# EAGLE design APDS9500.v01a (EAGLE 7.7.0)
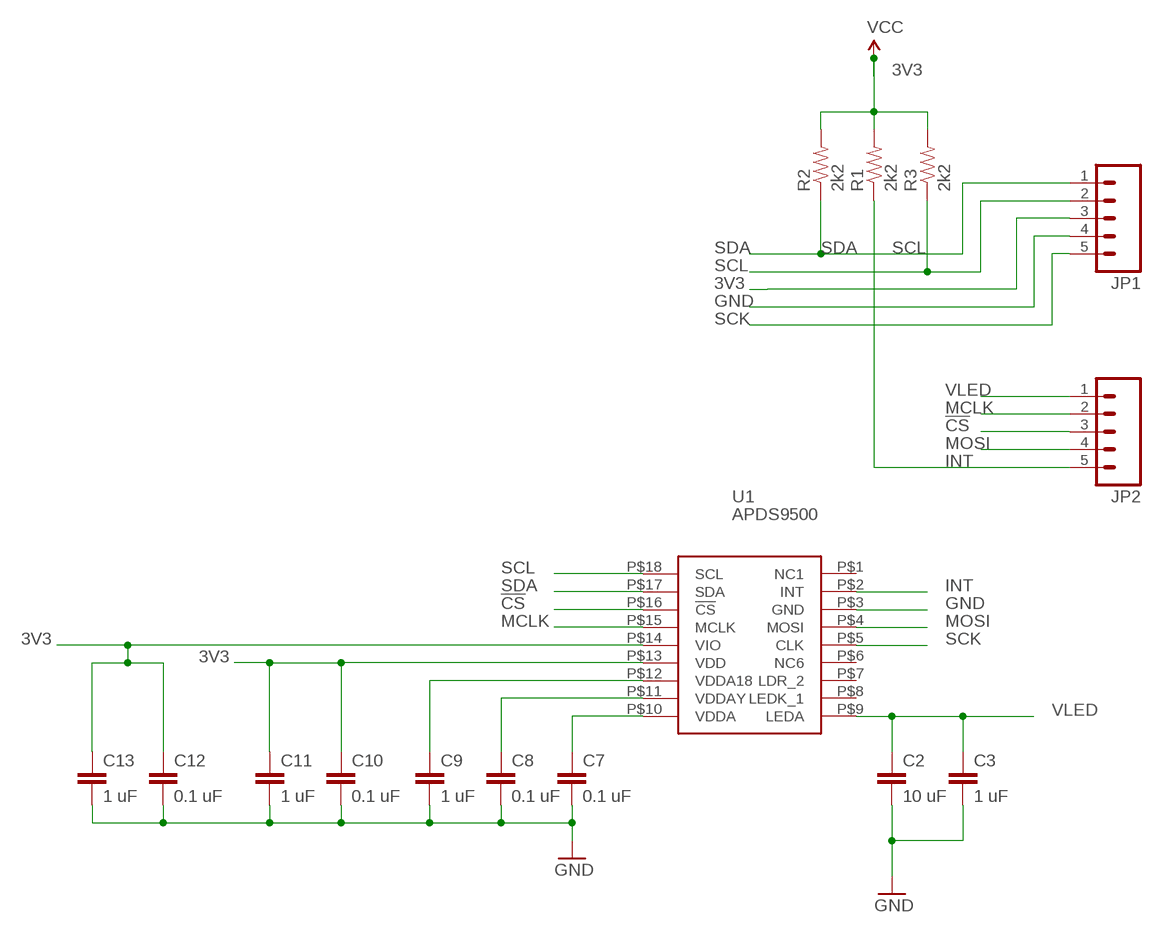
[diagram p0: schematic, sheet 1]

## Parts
C2  10 uF  CAP0402-CAP  [0402-CAP]
C3  1 uF  CAP0402-CAP  [0402-CAP]
C7  0.1 uF  CAP0402-CAP  [0402-CAP]
C8  0.1 uF  CAP0402-CAP  [0402-CAP]
C9  1 uF  CAP0402-CAP  [0402-CAP]
C10  0.1 uF  CAP0402-CAP  [0402-CAP]
C11  1 uF  CAP0402-CAP  [0402-CAP]
C12  0.1 uF  CAP0402-CAP  [0402-CAP]
C13  1 uF  CAP0402-CAP  [0402-CAP]
JP1  M05NO_SILK  [1X05_NO_SILK]
JP2  M05NO_SILK  [1X05_NO_SILK]
R1  2k2  0402RES.KW  [0402-RES]
R2  2k2  0402RES.KW  [0402-RES]
R3  2k2  0402RES.KW  [0402-RES]
U1  APDS9500  [APDS9500]

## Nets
3V3: C10.1 C11.1 C12.1 C13.1 JP1.3 R1.2 R2.2 R3.2 U1.P$13(VDD) U1.P$14(VIO) ; supply symbol labelled VCC
!CS: JP2.3 U1.P$16(!CS)
GND: C2.2 C3.2 C7.2 C8.2 C9.2 C10.2 C11.2 C12.2 C13.2 JP1.4 U1.P$3(GND)
INT: JP2.5 R1.1 U1.P$2(INT)
MCLK: JP2.2 U1.P$15(MCLK)
MOSI: JP2.4 U1.P$4(MOSI)
N$1: C7.1 U1.P$10(VDDA)
N$2: C8.1 U1.P$11(VDDAY)
N$4: C9.1 U1.P$12(VDDA18)
SCK: JP1.5 U1.P$5(CLK)
SCL: JP1.2 R3.1 U1.P$18(SCL)
SDA: JP1.1 R2.1 U1.P$17(SDA)
VLED: C2.1 C3.1 JP2.1 U1.P$9(LEDA)
Unconnected: U1.P$1(NC1) U1.P$6(NC6)

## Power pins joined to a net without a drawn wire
LDR_2: U1.P$7(LDR_2)
LEDK_1: U1.P$8(LEDK_1)

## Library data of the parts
C2 C3 C7-C13 = SparkFun-Capacitors:CAP: Capacitor
JP1 JP2 = SparkFun-Connectors:M05: Header 5 Standard 5-pin 0.1" header. Use with straight break away headers (SKU : PRT-00116), right angle break away headers (PRT-00553), swiss pins (PRT-00743), machine pins (PRT-00117), and female headers (PRT-00115). Molex polarized connector foot print use with SKU : PRT-08230 with associated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
R1-R3 = SparkFun-Resistors:0402RES.KW
U1 = kris:APDS9500: APDS-9500 Broadcom proximity sensor, gesturedetection sensor, camera https://www.broadcom.com/products/optical-sensors/proximity-sensors/apds-9500#overview

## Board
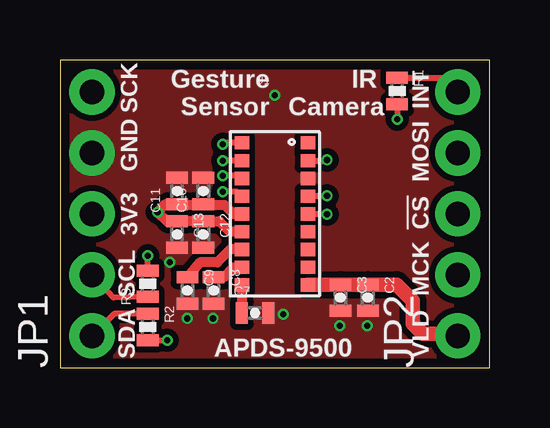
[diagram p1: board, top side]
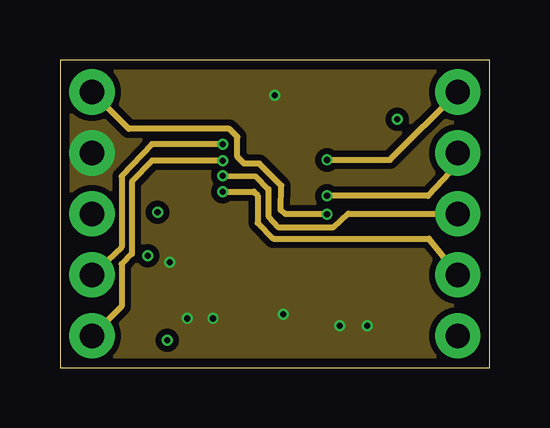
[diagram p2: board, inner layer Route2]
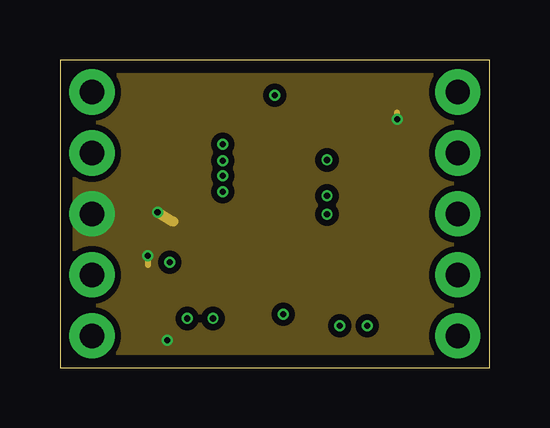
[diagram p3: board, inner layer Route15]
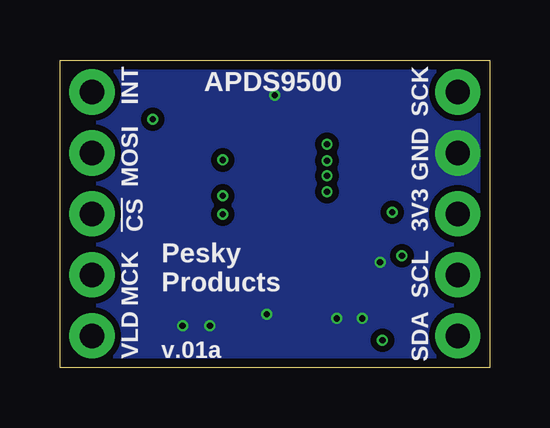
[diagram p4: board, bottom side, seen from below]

Size 17.91 x 12.83 mm. Coordinates in mm from the lower left corner, seen from the top.
Outline: 0,0 17.91,0 17.91,12.83 0,12.83 0,0
Copper layers (1*2*15*16): Top 0.035559375mm / dielectric 0.17018125mm / Route2 0.01778125mm / dielectric 47mil / Route15 0.01778125mm / dielectric 0.17018125mm / Bottom 0.035559375mm
Design rules "OSHPark-4layer *": minimum track width 5mil, minimum drill 10mil, track to track 5mil, track to pad 5mil, pad to pad 5mil, via to via 5mil, smd to smd 5mil, copper to edge 15mil, drill to drill 6mil, minimum pad ring 4mil, minimum via ring 4mil, stop-mask expansion 2.5mil, vias tented up to drill 20mil, thermal gap 10mil

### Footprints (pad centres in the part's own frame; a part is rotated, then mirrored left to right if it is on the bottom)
0402-CAP = smd 0.5 x 0.9: 1 -0.55,0; 2 0.55,0
1X05_NO_SILK = drill 1.016 pad 1.88: 1 0,0; 2 2.54,0; 3 5.08,0; 4 7.62,0; 5 10.16,0
0402-RES = smd 0.5 x 0.9: 1 -0.55,0; 2 0.55,0
APDS9500 = smd 0.6 x 0.55: P$1 1.377,2.96; P$2 1.377,2.22; P$3 1.377,1.48; P$4 1.377,0.74; P$5 1.377,0; P$6 1.377,-0.74; P$7 1.377,-1.48; P$8 1.377,-2.22; P$9 1.377,-2.96; P$10 -1.377,-2.96; P$11 -1.377,-2.22; P$12 -1.377,-1.48; P$13 -1.377,-0.74; P$14 -1.377,0; P$15 -1.377,0.74; P$16 -1.377,1.48; P$17 -1.377,2.22; P$18 -1.377,2.96

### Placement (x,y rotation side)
C2  12.83,2.92 270 top
C3  11.68,2.92 270 top
C7  8.13,2.29 0 top
C8  6.4,3.23 270 top
C9  5.31,3.23 270 top
C10  5.97,7.37 90 top
C11  4.88,7.37 90 top
C12  5.97,5.56 270 top
C13  4.88,5.56 270 top
JP1  1.33,1.33 90 top
JP2  16.57,1.33 90 top
R1  14.05,11.53 270 top
R2  3.66,1.7 270 top
R3  3.66,3.51 90 top
U1  8.95,6.41 0 top

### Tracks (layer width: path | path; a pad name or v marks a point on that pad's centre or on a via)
3V3  (via drill 0.25)
  Top 0.203: 14.05,10.26 v14.05,10.36
  Top 0.254: R2.2 4.41,1.15 v4.47,1.15 | R3.2 v3.66,4.67 | R1.2 v14.05,10.36
  Top 0.406: U1.P$14 7.23,6.41 6.86,6.78 5.93,6.78 | 5.93,6.78 C10.1 | U1.P$13 7.56,5.69 7.06,5.69 6.64,6.11 C12.1 C13.1 4.66,6.09 4.48,6.09 v4.06,6.48 4.38,6.82 C11.1 4.91,6.78 5.93,6.78
  Route15 0.254: v4.47,1.15 4.45,1.09 | v3.66,4.67 3.66,4.29 | v14.05,10.36 14.05,10.64
  Route15 0.406: v4.06,6.48 4.72,6.1
  pour Route15 (isolate 0.254, no thermals): 0.64,12.19 17.27,12.19 17.27,0.64 0.64,0.64
!CS  (via drill 0.25)
  Top 0.254: U1.P$16 7.35,8 v6.78,8
  Route2 0.254: v6.78,8 8.15,7.98 8.69,7.44 8.69,6.33 9.09,5.87 11.4,5.87 12.01,6.43 16.56,6.43 JP2.3 16.56,6.53
GND  (via drill 0.25)
  Route2 0.254: 1.68,8.61 JP1.4
  other vias: 9.3,2.24 11.66,1.75 12.8,1.75 6.38,2.06 5.31,2.06 4.57,4.39 8.95,11.35
  pour Top (isolate 0.254, no thermals): 0.05,12.8 17.98,12.8 17.98,0 0,0 0,12.83
  pour Route2 (isolate 0.254, no thermals): 0.03,12.93 17.96,12.93 17.96,0.13 -0.03,0.13 -0.03,12.95
  pour Bottom (isolate 0.254, no thermals): 0.03,12.8 17.96,12.8 17.96,0 -0.03,0 -0.03,12.83
INT  (via drill 0.25)
  Top 0.254: U1.P$2 11.12,8.63 v11.12,8.66 | R1.1 15.98,12.08 JP2.5
  Route2 0.254: v11.12,8.66 13.74,8.66 JP2.5
MCLK  (via drill 0.25)
  Top 0.254: U1.P$15 7.38,7.33 v6.78,7.34
  Route2 0.254: 16.51,4.29 16.51,3.94 JP2.2 15.37,5.38 8.89,5.38 8.23,6.04 8.23,7.19 8.08,7.34 v6.78,7.34
MOSI  (via drill 0.25)
  Top 0.254: U1.P$4 10.53,7.16 v11.12,7.16
  Route2 0.254: 16.56,9.09 16.56,8.97 | 16.56,8.97 16.56,8.46 15.34,7.16 v11.12,7.16 | JP2.4 16.56,8.97
N$1
  Top 0.406: U1.P$10 C7.1
N$2
  Top 0.406: C8.1 6.82,3.78 7.21,4.19 U1.P$11
N$4
  Top 0.406: U1.P$12 7.09,4.93 6.55,4.39 5.83,4.39 C9.1
SCK  (via drill 0.25)
  Top 0.254: U1.P$5 11.11,6.41 v11.12,6.4
  Route2 0.254: v11.12,6.4 9.4,6.4 9.2,6.58 9.22,7.59 8.31,8.51 7.67,8.51 7.39,8.79 7.39,9.63 7.06,9.96 2.87,9.96 JP1.5
SCL  (via drill 0.25)
  Top 0.254: U1.P$18 6.83,9.37 v6.78,9.32 | R3.1 2.23,2.93 JP1.2
  Route2 0.254: v6.78,9.32 3.83,9.32 2.56,7.98 2.56,5.03 JP1.2
SDA  (via drill 0.25)
  Top 0.254: U1.P$17 v6.78,8.63 v6.78,8.64 | R2.1 2.25,2.25 JP1.1
  Route2 0.254: v6.78,8.64 3.83,8.64 3,7.75 3,4.75 2.56,4.32 2.56,2.56 JP1.1
VLED
  Top 0.406: 11.67,3.45 C3.1 | 16.54,1.42 JP2.1
  Top 0.61: U1.P$9 11.67,3.45 | C3.1 C2.1 14.03,3.47 14.71,2.79 14.71,1.83 15.11,1.42 16.54,1.42

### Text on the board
tPlace: Gesture / Sensor | IR / Camera | SCK | INT | GND | MOSI | 3V3 | !CS | SCL | MCK | APDS-9500 | SDA | VLD
bPlace: SCK | INT | APDS9500 | GND | MOSI | 3V3 | !CS | SCL | MCK | Pesky / Products | SDA | VLD | v.01a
